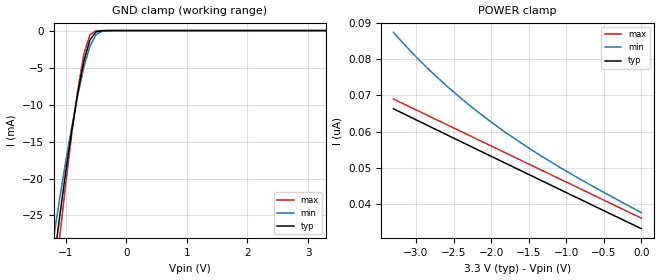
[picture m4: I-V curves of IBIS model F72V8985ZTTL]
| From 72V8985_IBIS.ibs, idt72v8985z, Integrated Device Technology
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|   Model F72V8985ZTTL
[Model]   F72V8985ZTTL
Model_type   Input
Vinl =  0.000V
Vinh =  3.000V
Vmeas =  1.500V
C_comp   3.00pF   NA   NA
[Temperature Range]   25.00   85.00   -40.00
[Voltage Range]   3.30V   3.00V   3.60V
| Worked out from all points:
|   GND clamp passes 1 mA (typ) near -0.57 V on its own axis
[GND_clamp]
| voltage   I(typ)   I(min)   I(max)
-3.3V     -192mA     -165mA     -219mA
-1.2V     -31.63mA   -28.05mA   -35.76mA
-1.1V     -25.24mA   -22.77mA   -28.08mA
-1V       -19.19mA   -17.76mA   -20.79mA
-900mV    -13.56mA   -13.06mA   -14.03mA
-800mV    -8.467mA   -8.749mA   -8.014mA
-700mV    -4.18mA    -4.989mA   -3.207mA
-600mV    -1.277mA   -2.121mA   -567uA
-500mV    -181uA     -556uA     -33.75uA
-400mV    -14.85uA   -87.38uA   -1.156uA
-300mV    -894nA     -10.41uA   -28.92nA
3.3V      33.07nA    40.87nA    33nA
[POWER_clamp]
| voltage   I(typ)   I(min)   I(max)
-3.3V     66.3nA     87.45nA    69nA
-3V       63.25nA    80.73nA    66nA
-2.6V     59.2nA     72.78nA    62nA
-2.3V     56.17nA    67.47nA    59nA
-1.9V     52.14nA    61.12nA    55nA
-1.5V     48.11nA    55.44nA    51nA
-1.1V     44.1nA     50.26nA    47nA
-600mV    39.08nA    44.29nA    42nA
0V        33.09nA    37.53nA    36nA
